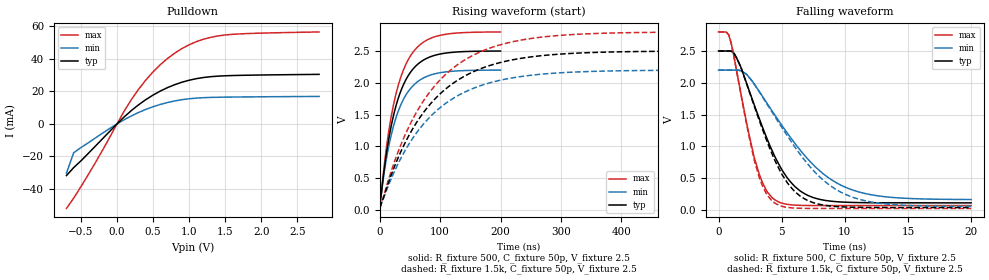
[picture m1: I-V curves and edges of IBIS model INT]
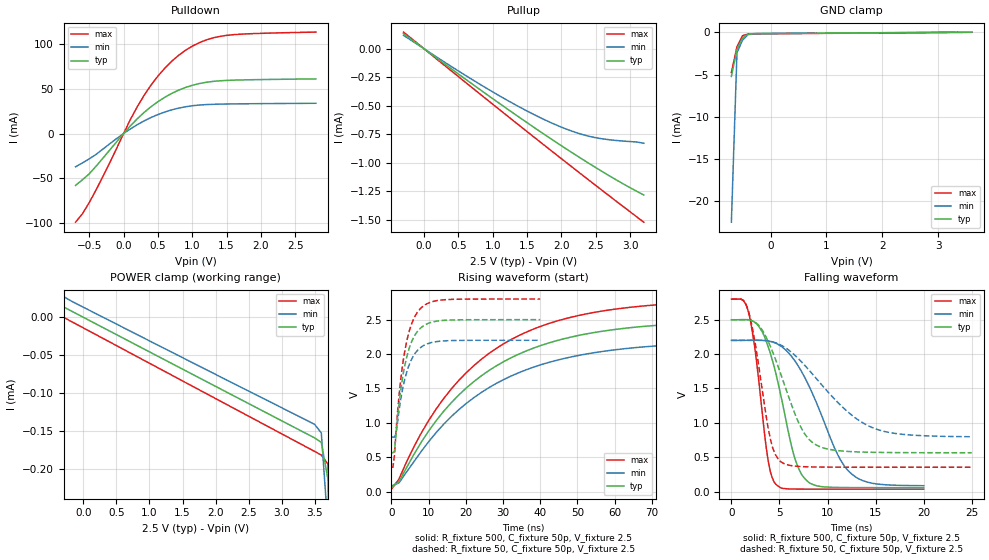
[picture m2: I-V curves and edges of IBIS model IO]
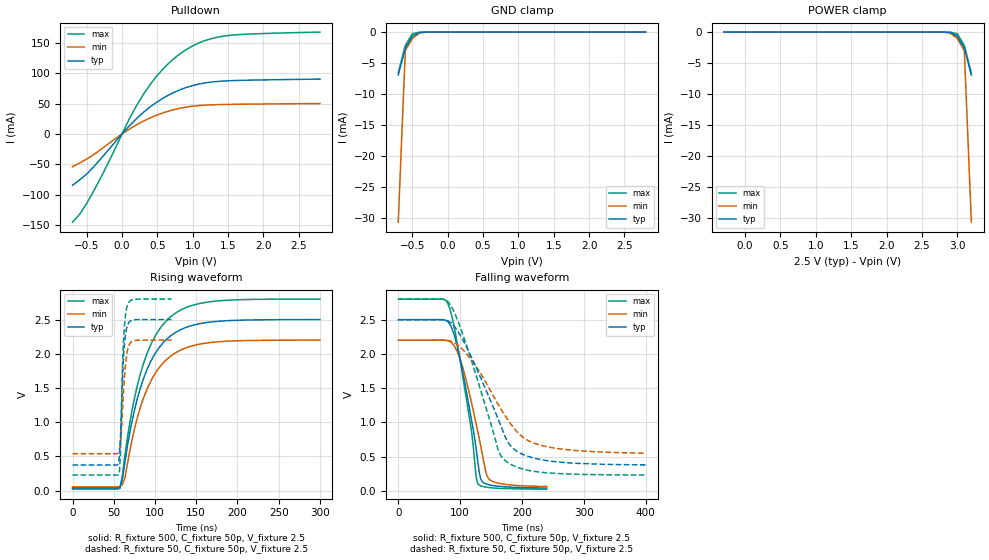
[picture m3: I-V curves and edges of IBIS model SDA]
[IBIS Ver]   3.2
[Comment Char]   |_char
| VDD Nom: 2.5v, Min: 2.2v, Max: 2.8v
[File name]   pca9674_2_5v.ibs
[File Rev]   1
[Date]   08-25-2008
[Source]
[Notes]
[Disclaimer]
(C) Copyright 2007 NXP Semiconductors
All rights reserved
NXP Semiconductors (NXP) does not warrant that this model and any other
accompanying information (Model) accurately or fully represents the
operating characteristics and specifications of the semiconductor
products to which the Model relates.  Moreover, the Model is furnished
on an "as is" and with "all faults" basis, and without support or
warranty of any kind.  NXP disclaims all warranties, whether expressed
or implied or statutory, including without limitation all implied
warranties of non-infringement, merchantability and fitness for any
purpose, and those arising from a course of dealing or usage of trade.
NXP does not convey any license under its or any third party's patents,
copyrights or other intellectual property or proprietary rights.
You and your company assume any and all risks and liability arising out
of the application or use of the Model.
In no event shall NXP be liable for any direct, indirect, special,
consequential or incidental damages, however caused, whether in
warranty, contract or tort (including negligence), strict liability or
other legal theory, including, without limitation, for lost profits,
business interruption, or corruption or loss of data or information,
arising out of or in connection with the use of or the inability to use
the Model, even if NXP has been advised of the possibility of such
damages.
NXP provides the Model as a courtesy to our customers. You and your
company shall not distribute, convey, sell, or give the Model to anyone
else without receiving prior written permission from NXP.
NXP reserves the right to make changes without notice to the Model to
improve reliability, function, or design.
Please be aware that your receipt and subsequent use of the Model shall
serve as acceptance of these terms and conditions.  If you do not
accept these terms, return or destroy the Model immediately.
[Copyright]
2008
| SO16 package
[Component]   PCA9674D
Si_location Pin
Timing_location Pin
[Manufacturer]   NXP Semiconductors
[Package]
R_pkg   1.75E-01   1.28E-01   2.11E-01
L_pkg   5.03E-09   3.94E-09   6.26E-09
C_pkg   0.794p   0.715p   0.869p
[Pin] signal_name   model_name   R_pin   L_pin   C_pin
1   AD0   ADDR   1.99E-01  6.26E-09  8.22E-13
2   AD1   ADDR   2.11E-01  5.46E-09  8.69E-13
3   AD2   ADDR   1.56E-01  4.44E-09  7.60E-13
4   P0   IO   1.28E-01  3.94E-09  7.17E-13
5   P1   IO   1.28E-01  3.94E-09  7.15E-13
6   P2   IO   1.56E-01  4.44E-09  7.60E-13
7   P3   IO   2.11E-01  5.46E-09  8.69E-13
8   VSS   GND   1.99E-01  6.26E-09  8.43E-13
9   P4   IO   1.99E-01  6.26E-09  8.43E-13
10   P5   IO   2.11E-01  5.46E-09  8.69E-13
11   P6   IO   1.56E-01  4.44E-09  7.60E-13
12   P7   IO   1.28E-01  3.94E-09  7.17E-13
13   INTb   INT   1.28E-01  3.94E-09  7.15E-13
14   SCL   SCL   1.56E-01  4.44E-09  7.60E-13
15   SDA   SDA   2.11E-01  5.46E-09  8.69E-13
16   VDD   POWER   1.99E-01  6.26E-09  8.43E-13
| TSSOP16 package
[Component]   PCA9674PW
Si_location Pin
Timing_location Pin
[Manufacturer]   NXP Semiconductors
[Package]
R_pkg   3.95E-02   3.52E-02   4.56E-02
L_pkg   1.94n   1.65n   2.40n
C_pkg   .446p   .335p   .771p
[Pin] signal_name   model_name   R_pin   L_pin   C_pin
1   AD0   ADDR   3.52E-02  2.40E-09  4.36E-13
2   AD1   ADDR   3.70E-02  1.93E-09  4.38E-13
3   AD2   ADDR   4.56E-02  1.76E-09  3.45E-13
4   P0   IO   4.00E-02  1.65E-09  3.35E-13
5   P1   IO   4.00E-02  1.65E-09  3.35E-13
6   P2   IO   4.56E-02  1.76E-09  3.45E-13
7   P3   IO   3.70E-02  1.93E-09  4.38E-13
8   VSS   GND   3.52E-02  2.40E-09  4.52E-13
9   P4   IO   3.52E-02  2.40E-09  4.52E-13
10   P5   IO   3.70E-02  1.93E-09  4.38E-13
11   P6   IO   4.56E-02  1.76E-09  3.45E-13
12   P7   IO   4.00E-02  1.65E-09  7.71E-13
13   INTb   ADDR   4.00E-02  1.65E-09  7.71E-13
14   SCL   SCL   4.56E-02  1.76E-09  3.45E-13
15   SDA   SDA   3.70E-02  1.93E-09  4.38E-13
16   VDD   POWER   3.52E-02  2.40E-09  4.52E-13
[Define Package Model]  HVQFN16
[Manufacturer]  ST-NXP Wireless
[OEM]  Unknown
[Description]  Full package model
|[Simulated] Chris Hunat
|[Approved] Wayne Nunn, Roger Real
[Number Of Pins]  16
[Pin Numbers]
|Pin Num   Terminal Name
1   | lead1:pin1
2   | lead2:pin2
3   | lead3:pin3
4   | lead4:pin4
5   | lead5:pin5
6   | lead6:pin6
7   | lead7:pin7
8   | lead8:pin8
9   | lead9:pin9
10   | lead10:pin10
11   | lead11:pin11
12   | lead12:pin12
13   | lead13:pin13
14   | lead14:pin14
15   | lead15:pin15
16   | lead16:pin16
[Model Data]
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[End Model Data]
[End Package Model]
| Models and submodels in the file (5): INT (Open_drain), IO (I/O), SDA (I/O_open_drain), SCL (Input), ADDR (Input)
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[Model]   INT
Model_type Open_drain
Vref=2.5
Vmeas=1.25
Rref=1.6k
Cref=50p
C_comp   5.2p   5p   5.4p
[Temperature Range] 27   85   -40
[Voltage Range]   2.5   2.2   2.8
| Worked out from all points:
|   slope of the pulldown table from 0 to 0.375 V, typ, clamps not added: 26.5 ohm
|   falling waveform, R_fixture 500, C_fixture 50p, V_fixture 2.5: 20-80 % time 2.99ns typ, 4.82ns min, 1.77ns max; typ from 2.5 V to 0.111 V
|   falling waveform, R_fixture 1.5k, C_fixture 50p, V_fixture 2.5: 20-80 % time 2.93ns typ, 4.7ns min, 1.75ns max; typ from 2.5 V to 0.037 V
|   rising waveform, R_fixture 500, C_fixture 50p, V_fixture 2.5: 20-80 % time 35.2ns typ, 35.2ns min, 35.1ns max; typ from 0.111 V to 2.5 V
|   rising waveform, R_fixture 1.5k, C_fixture 50p, V_fixture 2.5: 20-80 % time 106ns typ, 106ns min, 105ns max; typ from 0.037 V to 2.5 V
[Pulldown]
-700mV    -31.75mA   -30.26mA   -51.97mA
-600mV    -26.85mA   -17.73mA   -45.61mA
-200mV    -9.108mA   -5.667mA   -16.14mA
100mV     4.32mA     2.592mA    7.881mA
300mV     11.78mA    7.059mA    21.34mA
500mV     17.74mA    10.57mA    32mA
600mV     20.2mA     11.99mA    36.4mA
800mV     24.13mA    14.15mA    43.52mA
1.1V      27.83mA    15.88mA    50.58mA
1.4V      29.38mA    16.4mA     54.09mA
1.8V      29.94mA    16.61mA    55.54mA
2.8V      30.47mA    16.91mA    56.54mA
[Falling Waveform]
R_fixture=500
C_fixture=50p
V_fixture=2.5
V_fixture_min=2.2
V_fixture_max=2.8
0s        2.5V       2.2V       2.8V
808.1ps   2.5V       2.2V       2.755V
1.616ns   2.315V     2.198V     1.997V
2.828ns   1.654V     1.982V     827.6mV
3.636ns   1.223V     1.739V     367.6mV
4.444ns   845.3mV    1.497V     161.2mV
6.465ns   298.2mV    941.7mV    71.97mV
10.1ns    120.9mV    352.4mV    68.27mV
13.54ns   111.7mV    200.5mV    68.26mV
20ns      111.2mV    163.5mV    68.26mV
[Falling Waveform]
R_fixture=1.5k
C_fixture=50p
V_fixture=2.5
V_fixture_min=2.2
V_fixture_max=2.8
0s        2.5V       2.2V       2.8V
808.1ps   2.5V       2.2V       2.755V
1.616ns   2.313V     2.198V     1.988V
2.828ns   1.636V     1.979V     785mV
3.636ns   1.186V     1.729V     314.5mV
4.444ns   786.5mV    1.475V     109.3mV
6.465ns   217.1mV    875mV      25.8mV
10.1ns    45.22mV    240.3mV    22.66mV
13.33ns   37.49mV    92.17mV    22.66mV
20ns      37mV       55.35mV    22.66mV
[Rising Waveform]
R_fixture=500
C_fixture=50p
V_fixture=2.5
V_fixture_min=2.2
V_fixture_max=2.8
0s        111.2mV    161.8mV    68.26mV
2.02ns    216.8mV    223.3mV    217.4mV
6.061ns   551.2mV    512.2mV    596.5mV
12.12ns   964mV      868.9mV    1.064V
22.22ns   1.468V     1.305V     1.634V
36.36ns   1.908V     1.686V     2.133V
52.53ns   2.187V     1.928V     2.447V
70.71ns   2.347V     2.067V     2.628V
96.97ns   2.446V     2.153V     2.739V
200ns     2.499V     2.199V     2.799V
[Rising Waveform]
R_fixture=1.5k
C_fixture=50p
V_fixture=2.5
V_fixture_min=2.2
V_fixture_max=2.8
0s        37mV       54.11mV    22.66mV
30.3ns    820.7mV    728.3mV    915mV
48.48ns   1.177V     1.04V      1.315V
66.67ns   1.457V     1.285V     1.631V
84.85ns   1.679V     1.479V     1.88V
109.1ns   1.903V     1.675V     2.131V
157.6ns   2.184V     1.922V     2.446V
212.1ns   2.346V     2.064V     2.628V
290.9ns   2.445V     2.152V     2.739V
600ns     2.499V     2.199V     2.799V
[Ramp]
R_load=1.6k
dV/dt_r   1.479E+0/1.965E-9   1.465E+0/2.160E-9   1.489E+0/1.726E-9
dV/dt_f   1.479E+0/1.846E-10   1.465E+0/3.362E-10   1.489E+0/8.768E-11
|[End   INT
| [End   IO
[Model]   IO
Model_type I/O
Vinh=1.5
Vinl=0.75
Vref=2.5
Vmeas=1.25
Rref=500
Cref=50p
C_comp   7p   6.8p   7.2p
[Model Spec]
Vinh   1.494   1.195   1.893
Vinl   1.023   0.854   1.563
[Temperature Range] 27   85   -40
[Voltage Range]   2.5   2.2   2.8
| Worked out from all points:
|   slope of the pulldown table from 0 to 0.375 V, typ, clamps not added: 13.3 ohm
|   slope of the pullup table from 0 to 0.375 V, typ, clamps not added: 2.25 kohm
|   GND clamp passes 1 mA (typ) near -0.52 V on its own axis
|   falling waveform, R_fixture 500, C_fixture 50p, V_fixture 2.5: 20-80 % time 2.41ns typ, 4ns min, 1.41ns max; typ from 2.5 V to 0.056 V
|   falling waveform, R_fixture 50, C_fixture 50p, V_fixture 2.5: 20-80 % time 3.12ns typ, 5.76ns min, 1.66ns max; typ from 2.5 V to 0.564 V
|   rising waveform, R_fixture 500, C_fixture 50p, V_fixture 2.5: 20-80 % time 28.7ns typ, 29.5ns min, 28ns max; typ from 0.055 V to 2.5 V
|   rising waveform, R_fixture 50, C_fixture 50p, V_fixture 2.5: 20-80 % time 3.52ns typ, 3.59ns min, 3.48ns max; typ from 0.564 V to 2.5 V
[Pullup]
-300mV    132.9uA    118uA      146.5uA
500mV     -221.6uA   -195uA     -244.5uA
1V        -438.3uA   -378.9uA   -487.1uA
1.5V      -648.9uA   -546.8uA   -727.5uA
1.9V      -811.8uA   -663.1uA   -918uA
2.2V      -929.9uA   -733.5uA   -1.06mA
2.5V      -1.044mA   -781.3uA   -1.2mA
2.9V      -1.186mA   -810.6uA   -1.386mA
3.2V      -1.284mA   -830uA     -1.523mA
[Pulldown]
-700mV    -57.71mA   -36.98mA   -98.68mA
-600mV    -51.44mA   -32.7mA    -89.33mA
-500mV    -44.74mA   -28.1mA    -76.78mA
-200mV    -18.1mA    -11.23mA   -32.15mA
100mV     8.746mA    5.272mA    15.89mA
300mV     23.67mA    14.2mA     42.8mA
500mV     35.58mA    21.22mA    64.11mA
800mV     48.34mA    28.35mA    87.14mA
1.1V      55.72mA    31.81mA    101.2mA
1.4V      58.81mA    32.83mA    108.3mA
1.8V      59.91mA    33.24mA    111.1mA
2.8V      60.93mA    33.79mA    113.1mA
[GND Clamp]
-700mV    -5.214mA   -22.45mA   -4.761mA
-600mV    -2.033mA   -2.422mA   -1.708mA
-500mV    -655.6uA   -909.6uA   -400.5uA
-400mV    -212.8uA   -276uA     -193uA
-200mV    -158.7uA   -141uA     -176.5uA
3.6V      13.62uA    27.33uA    109.1pA
[POWER Clamp]
-300mV    13.62uA    27.33uA    109.1pA
-100mV    4.551uA    17.65uA    -9.31uA
3.5V      -158.7uA   -141uA     -176.5uA
3.6V      -164.6uA   -152.1uA   -181.2uA
3.7V      -212.8uA   -276uA     -193uA
3.8V      -655.6uA   -909.6uA   -400.5uA
4V        -5.214mA   -22.45mA   -4.761mA
[Falling Waveform]
R_fixture=500
C_fixture=50p
V_fixture=2.5
V_fixture_min=2.2
V_fixture_max=2.8
0s        2.5V       2.2V       2.8V
1.818ns   2.499V     2.201V     2.589V
2.424ns   2.463V     2.201V     2.107V
3.838ns   2.104V     2.191V     436.2mV
4.646ns   1.707V     2.157V     102.3mV
6.465ns   546.4mV    1.928V     35.83mV
8.081ns   128.8mV    1.533V     34.45mV
10.91ns   59.6mV     580.2mV    34.05mV
12.53ns   57.13mV    252.8mV    34.02mV
20ns      55.55mV    84.44mV    34.01mV
[Falling Waveform]
R_fixture=50
C_fixture=50p
V_fixture=2.5
V_fixture_min=2.2
V_fixture_max=2.8
0s        2.5V       2.2V       2.8V
1.263ns   2.501V     2.2V       2.779V
1.768ns   2.5V       2.201V     2.632V
2.525ns   2.457V     2.201V     2.119V
4.04ns    2.119V     2.186V     774.4mV
5.051ns   1.745V     2.138V     442.8mV
7.323ns   911.6mV    1.883V     362.7mV
9.091ns   659.2mV    1.602V     355.9mV
14.9ns    569.9mV    917.3mV    353.7mV
25ns      564.3mV    797.1mV    353.7mV
[Rising Waveform]
R_fixture=500
C_fixture=50p
V_fixture=2.5
V_fixture_min=2.2
V_fixture_max=2.8
0s        55.5mV     81.08mV    34.01mV
2.02ns    145.4mV    125.5mV    180.6mV
6.061ns   541.7mV    435.7mV    652.6mV
10.1ns    887.5mV    731.6mV    1.041V
20.2ns    1.51V      1.285V     1.732V
32.32ns   1.95V      1.683V     2.215V
46.46ns   2.223V     1.936V     2.51V
62.63ns   2.374V     2.077V     2.67V
86.87ns   2.461V     2.161V     2.761V
200ns     2.5V       2.2V       2.8V
[Rising Waveform]
R_fixture=50
C_fixture=50p
V_fixture=2.5
V_fixture_min=2.2
V_fixture_max=2.8
0s        564.2mV    792.2mV    353.7mV
404ps     564.2mV    792.2mV    353.7mV
808.1ps   586.5mV    792.4mV    526.5mV
1.212ns   815.1mV    836.7mV    855.6mV
2.02ns    1.266V     1.169V     1.385V
3.636ns   1.843V     1.646V     2.057V
5.253ns   2.157V     1.904V     2.414V
7.677ns   2.37V      2.087V     2.655V
14.14ns   2.49V      2.191V     2.789V
40ns      2.5V       2.2V       2.8V
[Ramp]
R_load=500
dV/dt_r   2.854E-1/1.585E-9   2.173E-1/3.221E-9   3.507E-1/9.177E-10
dV/dt_f   1.467E+0/7.289E-10   1.271E+0/1.459E-9   1.660E+0/3.514E-10
|[End   IO
| [End   SDA
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[Model]   SDA
Model_type I/O_open_drain
Vinh=1.5
Vinl=0.75
Vref=2.5
Vmeas=1.25
Rref=1k
Cref=50p
C_comp   6p   5.8p   6.2p
[Model Spec]
[Temperature Range] 27   85   -40
[Voltage Range]   2.5   2.2   2.8
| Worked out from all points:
|   slope of the pulldown table from 0 to 0.375 V, typ, clamps not added: 8.82 ohm
|   GND clamp passes 1 mA (typ) near -0.52 V on its own axis
|   falling waveform, R_fixture 500, C_fixture 50p, V_fixture 2.5: 20-80 % time 29.1ns typ, 31.6ns min, 28.4ns max; typ from 2.5 V to 0.041 V
|   falling waveform, R_fixture 50, C_fixture 50p, V_fixture 2.5: 20-80 % time 60.6ns typ, 68.7ns min, 52.9ns max; typ from 2.5 V to 0.379 V
|   rising waveform, R_fixture 500, C_fixture 50p, V_fixture 2.5: 20-80 % time 35.4ns typ, 35.5ns min, 35.3ns max; typ from 0.037 V to 2.5 V
|   rising waveform, R_fixture 50, C_fixture 50p, V_fixture 2.5: 20-80 % time 4.34ns typ, 5.3ns min, 3.79ns max; typ from 0.374 V to 2.5 V
[Pulldown]
-700mV    -84.71mA   -54.07mA   -145.5mA
-600mV    -75.81mA   -47.97mA   -132.5mA
-400mV    -54.01mA   -34.18mA   -93.93mA
-200mV    -27.3mA    -16.82mA   -48.96mA
100mV     13.05mA    7.75mA     24.12mA
300mV     35.44mA    21.05mA    64.86mA
500mV     53.16mA    31.45mA    96.69mA
800mV     71.93mA    41.95mA    130.5mA
1.1V      82.63mA    47.01mA    150.8mA
1.4V      87.08mA    48.54mA    160.7mA
1.8V      88.74mA    49.21mA    164.8mA
2.8V      90.48mA    50.19mA    168mA
[GND Clamp]
-700mV    -6.935mA   -30.66mA   -6.593mA
-600mV    -2.591mA   -2.99mA    -2.148mA
-500mV    -653.7uA   -1.019mA   -278.6uA
-400mV    -54.45uA   -160.3uA   -7.607uA
-300mV    -1.471uA   -7.716uA   -80.08nA
2.8V      157.3pA    305.4pA    145.7pA
[POWER Clamp]
-300mV    157.3pA    305.4pA    145.7pA
2.8V      -1.471uA   -7.716uA   -80.08nA
2.9V      -54.45uA   -160.3uA   -7.607uA
3V        -653.7uA   -1.019mA   -278.6uA
3.1V      -2.591mA   -2.99mA    -2.148mA
3.2V      -6.935mA   -30.66mA   -6.593mA
[Falling Waveform]
R_fixture=500
C_fixture=50p
V_fixture=2.5
V_fixture_min=2.2
V_fixture_max=2.8
0s        2.5V       2.2V       2.8V
80ns      2.472V     2.193V     2.74V
99.39ns   1.951V     1.941V     1.942V
118.8ns   1.019V     1.274V     848.5mV
126.1ns   607.3mV    972.7mV    196.4mV
128.5ns   436.1mV    869.8mV    106.9mV
133.3ns   173.8mV    656.4mV    73.17mV
140.6ns   105.3mV    313.9mV    55.45mV
147.9ns   85.93mV    161mV      46.3mV
240ns     41.13mV    62.75mV    24.28mV
[Falling Waveform]
R_fixture=50
C_fixture=50p
V_fixture=2.5
V_fixture_min=2.2
V_fixture_max=2.8
0s        2.5V       2.2V       2.8V
72.73ns   2.499V     2.2V       2.799V
84.85ns   2.458V     2.187V     2.709V
96.97ns   2.323V     2.126V     2.469V
117.2ns   1.975V     1.924V     1.937V
161.6ns   1.047V     1.262V     590.7mV
177.8ns   705mV      1.029V     409.4mV
202ns     529.7mV    778.9mV    316.6mV
234.3ns   450mV      657mV      268.4mV
400ns     378.9mV    550.1mV    230.6mV
[Rising Waveform]
R_fixture=500
C_fixture=50p
V_fixture=2.5
V_fixture_min=2.2
V_fixture_max=2.8
0s        36.68mV    54.25mV    22.15mV
57.58ns   54.78mV    61.72mV    33.04mV
60.61ns   170.3mV    93.88mV    241.5mV
63.64ns   427.5mV    189.4mV    527.6mV
72.73ns   1.047V     777.1mV    1.209V
84.85ns   1.596V     1.313V     1.811V
100ns     2.001V     1.709V     2.255V
121.2ns   2.283V     1.986V     2.563V
169.7ns   2.468V     2.168V     2.765V
300ns     2.5V       2.2V       2.8V
[Rising Waveform]
R_fixture=50
C_fixture=50p
V_fixture=2.5
V_fixture_min=2.2
V_fixture_max=2.8
0s        374mV      540mV      228.7mV
55.76ns   413.9mV    557.3mV    231.5mV
56.97ns   521mV      604mV      294mV
58.18ns   798.5mV    699.6mV    550.7mV
60.61ns   1.636V     1.168V     1.825V
61.82ns   1.954V     1.448V     2.191V
64.24ns   2.289V     1.833V     2.566V
66.67ns   2.419V     2.052V     2.71V
73.94ns   2.495V     2.191V     2.795V
120ns     2.5V       2.2V       2.8V
[Ramp]
R_load=500
dV/dt_r   1.478E+0/1.583E-9   1.463E+0/2.880E-9   1.488E+0/9.563E-10
dV/dt_f   1.476E+0/2.825E-8   1.457E+0/3.507E-8   1.487E+0/2.413E-8
|[End   SDA
| [End   SCL
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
